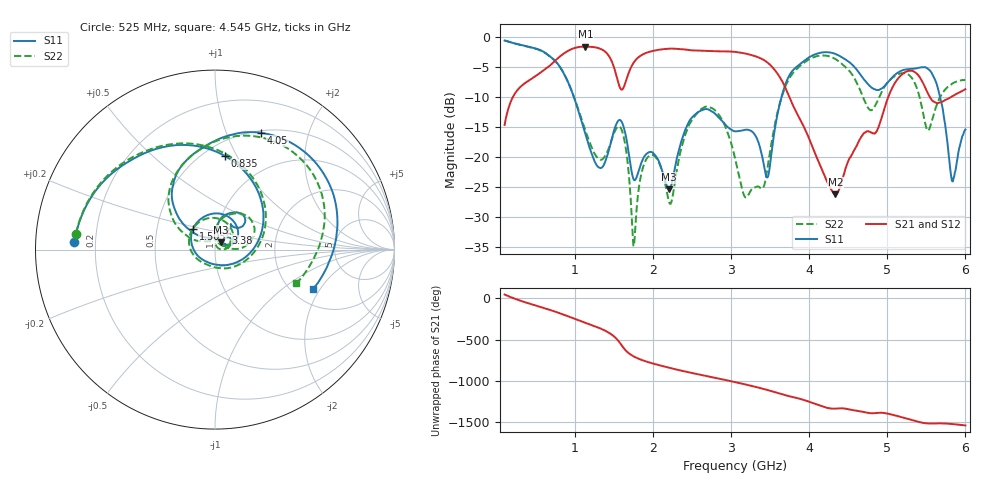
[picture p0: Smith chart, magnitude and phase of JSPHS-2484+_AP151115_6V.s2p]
!Mini-Circuits Laboratory
!S-Parameters
!Run/Lot/Date Code:MF33450/NA/1551
!Fixture/SN/Due: 90-4-20-21/70546/03/17/16
!Connection:PORT<IN> - pin<1>; PORT<OUT> - pin<7>;PORT<BIAS> - pin<4>;
!Tested With:PORT EXTENTION
!Network Analyzer:AG E5071C/74883/05/12/16
!Created: 01-07-2016 at 14:09:53
!MODEL: JSPHS-2484+
!S/N: V=6V
# MHZ S DB R 50
!Frequency  S11 dB  S11 DEG  S21 dB  S21 DEG  S12 dB  S12 DEG  S22 dB  S22 DEG
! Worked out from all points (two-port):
!   1181 points, 100 MHz to 6 GHz, reference 50 ohm
!   highest |S21| = -1.68 dB at 1.135 GHz (marker M1); lowest = -26.3 dB at 4.335 GHz (marker M2)
!   |S21| within 3 dB of the highest: 694 MHz to 1.489 GHz (794.6 MHz wide, 72.8 % of centre); 1.737 GHz to 3.497 GHz (1.761 GHz wide, 67.3 % of centre)
!   lowest |S11| = -25.4 dB at 2.205 GHz (marker M3), VSWR 1.11, Z = 53.4 + j4.38 ohm
!   |S11| at or under -10 dB: 984.9 MHz to 3.647 GHz (2.662 GHz wide, 115 % of centre); 5.675 GHz to end of sweep
!   |S22| runs from -34.9 to -0.7 dB; largest |S21 - S12| = 0.0016
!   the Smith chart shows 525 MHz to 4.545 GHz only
!   S11 on the Smith chart (normalised r, x): 525 MHz: 0.12, +0.03; 835 MHz: 0.63, +0.90; 1.505 GHz: 0.76, +0.18; 3.38 GHz: 1.11, +0.21; 4.05 GHz: 0.52, +1.33; 4.545 GHz: 2.56, -1.72
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100  -0.66 -44.7  -14.72 45.0  -14.71 45.0  -0.66 -44.6
525  -2.11 176.9  -6.33 -95.3  -6.33 -95.4  -2.15 173.6
835  -5.62 83.8  -3.05 168.9  -3.04 168.8  -5.64 80.2
1085  -14.09 -4.8  -1.70 81.2  -1.70 81.2  -13.74 -8.6
1135  -16.26 -23.3  -1.68 64.0  -1.68 64.0  -15.69 -28.2
1330  -21.88 -110.5  -2.07 -7.0  -2.06 -7.0  -20.51 -110.8
1505  -15.48 136.5  -5.32 -104.9  -5.31 -104.9  -15.97 153.4
1675  -18.18 21.6  -6.56 66.5  -6.56 66.5  -20.92 15.8
1755  -23.84 28.8  -4.30 15.2  -4.30 15.2  -34.90 47.3
2070  -20.63 20.0  -2.22 -88.0  -2.21 -88.0  -20.82 22.8
2205  -25.43 49.8  -2.03 -120.6  -2.03 -120.6  -27.50 38.2
2565  -12.71 63.4  -2.34 162.4  -2.34 162.4  -12.74 60.9
3050  -15.79 51.4  -2.56 65.4  -2.57 65.3  -20.27 2.4
3380  -18.96 56.8  -3.64 -8.2  -3.65 -8.3  -25.27 104.1
4035  -3.20 70.9  -18.15 175.7  -18.16 175.6  -3.56 72.7
4050  -3.10 68.4  -18.63 170.7  -18.64 170.6  -3.48 70.2
4335  -2.90 19.4  -26.27 104.1  -26.23 104.2  -3.75 20.0
4545  -4.62 -22.0  -19.66 88.8  -19.59 89.0  -6.23 -22.6
5020  -7.44 150.8  -9.81 40.7  -9.81 40.6  -7.40 115.1
5505  -5.23 20.4  -9.09 -74.1  -9.09 -74.1  -15.42 52.2
5830  -24.07 -0.3  -9.95 -82.0  -9.95 -81.9  -7.87 75.1
6000  -15.48 44.9  -8.77 -99.4  -8.77 -99.4  -7.25 62.2
